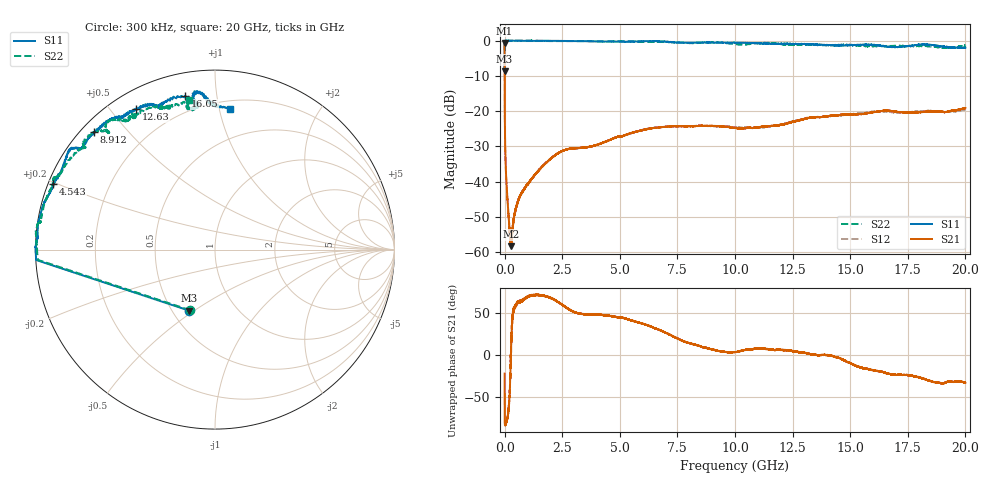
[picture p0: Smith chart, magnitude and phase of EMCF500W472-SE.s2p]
!EMCF500W472
!Johanson Technology Inc.
!www.johansontechnology.com
!Test Board Conditions:
!Substrate Type  RO4350B
!Substrate Thickness  6.6 mil
!Substrate Dk  3.66
!TL Type: GCPW
!TL Trace Width  13 mil
!TL Gap  7.5 mil
!PART MODE SINGLE ENDED (AKA BYPASS)
!DUT TOPOLOGY	SERIES-SHUNT
# MHz S  dB  R 50
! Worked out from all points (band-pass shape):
!   20001 points, 300 kHz to 20 GHz, reference 50 ohm
!   highest |S21| = -0.69 dB at 300 kHz (marker M1); lowest = -58.3 dB at 262.3 MHz (marker M2)
!   |S21| within 3 dB of the highest: start of sweep to 869.8 kHz
!   lowest |S11| = -8.7 dB at 300 kHz (marker M3), VSWR 2.17, Z = 30.4 - j24 ohm
!   |S11| at or under -10 dB: nowhere
!   |S22| runs from -8.8 to 0.0 dB; largest |S21 - S12| = 0.0051
!   S11 on the Smith chart (normalised r, x): 300 kHz: 0.61, -0.48; 4.543 GHz: 0.02, +0.19; 8.912 GHz: 0.03, +0.41; 12.63 GHz: 0.07, +0.58; 16.05 GHz: 0.11, +0.82; 20 GHz: 0.25, +1.08
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0.3  -8.66 -112.7  -0.69 -22.1  -0.65 -22.1  -8.75 -112.5
115.298  -0.00 179.7  -44.11 -76.0  -44.11 -76.4  -0.08 179.9
194.297  -0.01 179.1  -51.55 -59.8  -51.79 -58.5  -0.07 179.3
262.296  -0.01 179.0  -58.28 -6.9  -57.08 -10.6  -0.05 178.5
321.295  -0.01 178.7  -55.12 37.4  -55.13 35.5  -0.05 178.2
472.293  -0.03 178.0  -47.86 58.3  -47.86 58.1  -0.04 177.1
648.29  -0.05 177.3  -44.32 62.8  -44.40 63.6  -0.00 175.9
1339.28  -0.08 175.5  -37.82 71.7  -37.85 72.0  -0.04 171.5
2339.265  -0.07 167.4  -31.91 63.0  -31.87 62.5  -0.14 170.0
3334.25  -0.15 163.5  -30.40 49.1  -30.42 49.1  -0.13 163.9
4543.232  -0.26 158.0  -28.22 46.9  -28.22 46.7  -0.22 158.1
6667.2  -0.18 144.9  -24.66 30.5  -24.60 30.2  -0.37 150.8
8912.166  -0.51 135.8  -24.16 7.2  -24.20 7.2  -0.48 140.1
10000.15  -0.63 130.7  -24.73 3.4  -24.54 3.8  -1.02 132.5
12630.11  -0.93 119.2  -22.88 4.2  -22.73 3.9  -1.16 122.7
13334.1  -1.07 114.2  -21.82 0.3  -21.73 0.0  -1.22 120.8
14436.08  -1.33 111.6  -21.23 -2.9  -21.28 -2.9  -1.25 120.5
16047.06  -1.19 101.0  -20.26 -18.4  -20.10 -19.9  -1.55 107.8
16667.05  -1.78 97.1  -19.87 -22.2  -20.20 -23.1  -1.52 110.1
17367.04  -1.66 97.8  -20.35 -23.8  -20.41 -22.5  -1.55 109.1
18617.02  -1.30 94.6  -20.13 -32.2  -19.94 -33.2  -1.74 97.3
20000  -2.02 84.0  -19.11 -33.0  -19.41 -32.0  -1.46 99.7
